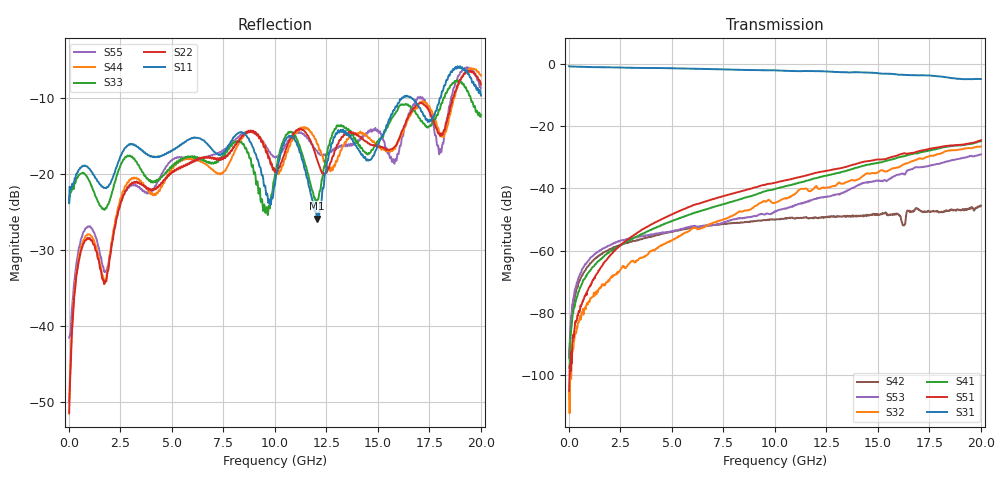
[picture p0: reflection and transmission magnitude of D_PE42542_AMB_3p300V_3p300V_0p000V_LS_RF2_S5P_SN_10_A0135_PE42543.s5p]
! Device ID: PE42542
! Device ID: PE42542
! File Path: z:\PE42542\PE42543_20140723_inv\AMB\3p300\LS_RF2\PE42542_AMB_3p300V_3p300V_0p000V_LS_RF2_S5P_SN_10_A0135_PE42543.s5p
! Serial: 10
! Lot: A0135_PE42543
! Temp: AMB
! VDD: 3.300
! VSS: 0.000
! Control_Hi: 3.300
! Control_Lo: 0.000
! Logic State: LS_RF2
! Port 1: RFC
! Port 2: RF1
! Port 3: RF2
! Port 5: RF3
! Port 6: RF4
! ThroughPath:1-3
! IDD: -0.000136019593
! ISS: 1.57066081e-010
#  Hz  S  RI  R  50
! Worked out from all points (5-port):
!   801 points, 10 MHz to 20 GHz, reference 50 ohm
!   strongest paths, dB at 10 MHz, 5.008 GHz, 10.01 GHz, 15 GHz, 20 GHz:
!     S31: -0.7, -1.4, -2.1, -3.0, -4.8
!     S51: -105.1, -48.3, -38.2, -30.7, -24.5
!     S41: -97.8, -50.5, -40.2, -31.8, -24.8
!     S32: -105.4, -56.7, -44.6, -34.9, -26.5
!     S53: -94.7, -53.8, -47.4, -37.5, -29.1
!     S42: -94.2, -53.9, -50.1, -48.6, -45.6
!   lowest |S11| = -25.8 dB at 12.05 GHz (marker M1), VSWR 1.11, Z = 52 + j4.82 ohm
!   |S11| at or under -10 dB: start of sweep to 16.16 GHz; 16.66 GHz to 18 GHz (1.348 GHz wide, 7.78 % of centre)
